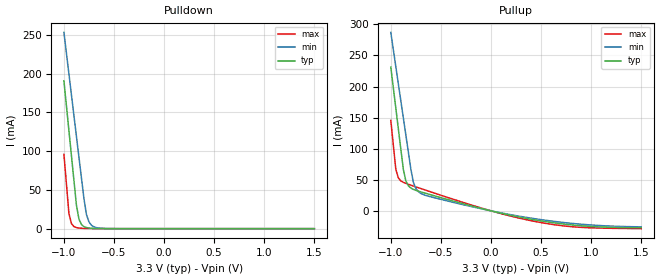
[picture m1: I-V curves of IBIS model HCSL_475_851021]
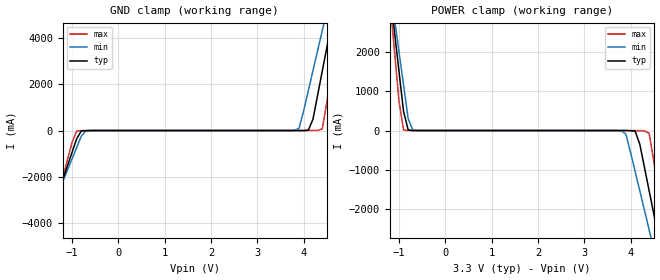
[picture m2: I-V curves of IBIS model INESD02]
|   This file is an IBIS representation of the   |
|   Integrated Circuit Systems, Inc.   |
|   ICS851021   |
[IBIS Ver]   4.0
[File name]   851021_rref_475.ibs
[File Rev]   1.0
[Date]   Dec 29 2006 | Last modified
|   Dec 29 2006 | Generated
[Source] Originated at Integrated Device Technology, Inc.
[Disclaimer]
IDT hereby grants the user of this IBIS model a non-exclusive,
nontransferable license to use this IBIS model under the following terms.
Before using this IBIS model, the user should read this license.
If the user does not accept these terms,  the IBIS model should be
returned to IDT within 30 days.
   The user is granted this license only to use the IBIS model and
is not granted rights to sell, load, rent, lease or license the IBIS
model in whole or in part, or in modified form to anyone other than
user. User may modify the IBIS model to suit its specific
applications but rights to derivative works and such modifications
shall belong to ICS.
   This IBIS model is provided on an "AS IS" basis and IDT makes
absolutely no warranty with respect to the information contained
herein. IDT DISCLAIMS AND CUSTOMER WAIVES ALL WARRANTIES, EXPRESS
OR IMPLIED, INCLUDING WARRANTIES OF MERCHANTABILITY OR FITNESS FOR
A PARTICULAR PURPOSE. The entire risk as to quality and performance
is with the Customer. ACCORDINGLY, IN NO EVENT SHALL THE COMPANY BE
LIABLE FOR ANY DAMAGES, WHETHER IN CONTRACT OR TORT,INCLUDING ANY
LOST PROFITS OR OTHER INCIDENTAL, CONSEQUENTIAL, EXEMPLARY, OR
PUNITIVE DAMAGES ARISING OUT OF THE USE OR APPLICATION OF THE IBIS
model provided in this package. Further, IDT reserves the right to
make changes without notice to any product herein to improve
reliability, function, or design. IDT does not convey any license
under patent rights or any other intellectual property rights,
including those of third parties.
   IDT is not obligated to provide maintenance or support
for the licensed IBIS model.
[Copyright]   Copyright 2006 by Integrated Device Technology, Inc.
[Component]   ICS851021AY
[Manufacturer] Integrated Device Technology, Inc.
[Package]
|TQFP 64 Pin lead+wire
|   typ   min   max
R_pkg   73.35m   65.90m   80.80m
L_pkg   2.615n   2.25n   2.98n
C_pkg   0.382p   0.366p   0.397p
[Pin] signal_name   model_name   R_pin   L_pin   C_pin
1   Q3   HCSL_475_851021   80.80m   2.98n   0.366p
2   nQ3   HCSL_475_851021   79.00m   2.81n   0.397p
3   VDD   POWER   74.90m   2.66n   0.390p
4   Q4   HCSL_475_851021   71.70m   2.54n   0.390p
5   nQ4   HCSL_475_851021   69.30m   2.44n   0.378p
6   GND   GND   67.60m   2.36n   0.373p
7   Q5   HCSL_475_851021   65.90m   2.30n   0.371p
8   nQ5   HCSL_475_851021   65.90m   2.25n   0.379p
9   VDD   POWER   65.90m   2.25n   0.379p
10   Q6   HCSL_475_851021   65.90m   2.30n   0.371p
11   nQ6   HCSL_475_851021   67.60m   2.36n   0.373p
12   Q7   HCSL_475_851021   69.30m   2.44n   0.378p
13   nQ7   HCSL_475_851021   71.70m   2.54n   0.390p
14   VDD   POWER   74.90m   2.66n   0.390p
15   Q8   HCSL_475_851021   79.00m   2.81n   0.397p
16   nQ8   HCSL_475_851021   80.80m   2.98n   0.366p
17   GND   GND   80.80m   2.98n   0.366p
|18  RREF   79.00m   2.81n   0.397p
19   Q9   HCSL_475_851021   74.90m   2.66n   0.390p
20   nQ9   HCSL_475_851021   71.70m   2.54n   0.390p
21   VDD   POWER   69.30m   2.44n   0.378p
22   Q10   HCSL_475_851021   67.60m   2.36n   0.373p
23   nQ10   HCSL_475_851021   65.90m   2.30n   0.371p
24   VDD   POWER   65.90m   2.25n   0.379p
25   VDDA   POWER   65.90m   2.25n   0.379p
|26  nc   65.90m   2.30n   0.371p
27   Q11   HCSL_475_851021   67.60m   2.36n   0.373p
28   nQ11   HCSL_475_851021   69.30m   2.44n   0.378p
29   VDD   POWER   71.70m   2.54n   0.390p
30   Q12   HCSL_475_851021   74.90m   2.66n   0.390p
31   nQ12   HCSL_475_851021   79.00m   2.81n   0.397p
32   GND   GND   80.80m   2.98n   0.366p
33   Q13   HCSL_475_851021   80.80m   2.98n   0.366p
34   nQ13   HCSL_475_851021   79.00m   2.81n   0.397p
35   VDD   POWER   74.90m   2.66n   0.390p
36   Q14   HCSL_475_851021   71.70m   2.54n   0.390p
37   nQ14   HCSL_475_851021   69.30m   2.44n   0.378p
38   Q15   HCSL_475_851021   67.60m   2.36n   0.373p
39   nQ15   HCSL_475_851021   65.90m   2.30n   0.371p
40   VDD   POWER   65.90m   2.25n   0.379p
41   Q16   HCSL_475_851021   65.90m   2.25n   0.379p
42   nQ16   HCSL_475_851021   65.90m   2.30n   0.371p
43   GND   GND   67.60m   2.36n   0.373p
44   Q17   HCSL_475_851021   69.30m   2.44n   0.378p
45   nQ17   HCSL_475_851021   71.70m   2.54n   0.390p
46   VDD   POWER   74.90m   2.66n   0.390p
47   Q18   HCSL_475_851021   79.00m   2.81n   0.397p
48   nQ18   HCSL_475_851021   80.80m   2.98n   0.366p
49   GND   GND   80.80m   2.98n   0.366p
50   CLK   INESD02   79.00m   2.81n   0.397p
51   nCLK   INESD02   74.90m   2.66n   0.390p
52   VDD   POWER   71.70m   2.54n   0.390p
53   Q19   HCSL_475_851021   69.30m   2.44n   0.378p
54   nQ19   HCSL_475_851021   67.60m   2.36n   0.373p
55   Q20   HCSL_475_851021   65.90m   2.30n   0.371p
56   nQ20   HCSL_475_851021   65.90m   2.25n   0.379p
57   VDD   POWER   65.90m   2.25n   0.379p
58   Q0   HCSL_475_851021   65.90m   2.30n   0.371p
59   nQ0   HCSL_475_851021   67.60m   2.36n   0.373p
60   Q1   HCSL_475_851021   69.30m   2.44n   0.378p
61   nQ1   HCSL_475_851021   71.70m   2.54n   0.390p
62   VDD   POWER   74.90m   2.66n   0.390p
63   Q2   HCSL_475_851021   79.00m   2.81n   0.397p
64   nQ2   HCSL_475_851021   80.80m   2.98n   0.366p
[Diff Pin]  inv_pin  vdiff tdelay_typ tdelay_min  tdelay_max
1   2   NA   0   0   0
4   5   NA   0   0   0
7   8   NA   0   0   0
10   11   NA   0   0   0
12   13   NA   0   0   0
15   16   NA   0   0   0
19   20   NA   0   0   0
22   23   NA   0   0   0
27   28   NA   0   0   0
30   31   NA   0   0   0
33   34   NA   0   0   0
36   37   NA   0   0   0
38   39   NA   0   0   0
41   42   NA   0   0   0
44   45   NA   0   0   0
47   48   NA   0   0   0
53   54   NA   0   0   0
55   56   NA   0   0   0
58   59   NA   0   0   0
60   61   NA   0   0   0
63   64   NA   0   0   0
|Input
50   51   NA   0   0   0
| Models and submodels in the file (2): HCSL_475_851021 (Output_ECL), INESD02 (Input)
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[Model]   HCSL_475_851021
Model_type  Output_ECL
Polarity   Non-Inverting
Vmeas = 0.3
Rref = 50
Cref = 0
Vref = 0
|Variable   typ   min   max
C_comp   2p   1.5p   2.5p
|Variable   typ   min   max
[Temperature Range]   25   0   70
|vddo
[Voltage Range]   3.3   3.135   3.465
|  Voltage   I(typ)   I(min)   I(max)
[Pullup]
-1V       231.3mA    287.2mA    145.6mA
-950mV    165.4mA    232.2mA    66.95mA
-925mV    132.5mA    204.7mA    53.21mA
-875mV    66.96mA    149.8mA    45.86mA
-850mV    48.22mA    122.3mA    44.19mA
-800mV    36.71mA    67.38mA    41.33mA
-775mV    34.58mA    46.1mA     39.96mA
-725mV    31.73mA    30.85mA    37.22mA
-250mV    10.23mA    8.861mA    12.13mA
475mV     -15.56mA   -13.58mA   -18.18mA
875mV     -23.69mA   -21.17mA   -26.35mA
1.5V      -27.26mA   -25.78mA   -28.68mA
[Pulldown]
-1V       190.7mA    253.2mA    96.06mA
-950mV    126.3mA    199.5mA    19.32mA
-925mV    94.15mA    172.6mA    6.574mA
-875mV    30.23mA    119mA      1.34mA
-850mV    12.34mA    92.17mA    792.6uA
-825mV    5.387mA    65.39mA    503.8uA
-800mV    2.598mA    38.64mA    322.7uA
-775mV    1.405mA    18.08mA    201.9uA
-750mV    838uA      8.675mA    122.1uA
-725mV    531uA      4.358mA    71.4uA
-550mV    17.95uA    128.7uA    737nA
1.5V      106.7pA    2.661nA    840.3fA
[Ramp]
|   typ   min   max
dV/dt_r   0.4V/0.2ns   0.35V/0.25ns   0.45V/0.2ns
dV/dt_f   0.4V/0.2ns   0.35V/0.25ns   0.45V/0.2ns
R_load =   50.0000
[Model]   INESD02
Model_type   Input
Polarity   Non-Inverting
Vinl = 1.4V
Vinh = 1.85V
|   typ   min   max
C_comp   2pF   1.5pF   2.5pF
|   typ   min   max
[Voltage range]  3.3V   3.15V   3.45V
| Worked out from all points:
|   GND clamp passes 1 mA (typ) near -0.60 V on its own axis
|   POWER clamp passes 1 mA (typ) near -0.70 V on its own axis
[GND_clamp]
|Voltage   I(typ)   I(min)   I(max)
-3.3V     -14.52A    -12.54A    -17.85A
-1.6V     -4.484A    -4.176A    -5.037A
-1.5V     -3.894A    -3.684A    -4.283A
-900mV    -353.5mA   -734.3mA   -21.75mA
-700mV    -3.477mA   -14.23mA   -2.542mA
3.9V      93.7uA     99.11mA    24.3nA
4.2V      488.4mA    2.584A     154.2uA
4.4V      2.557A     4.308A     69.78mA
4.6V      4.628A     6.034A     2.547A
4.7V      5.664A     6.897A     3.87A
4.8V      6.7A       7.76A      5.194A
6.6V      25.37A     23.32A     29.05A
[POWER_clamp]
|Voltage   I(typ)   I(min)   I(max)
-3.3V     25.37A     21.89A     31.23A
-1.2V     3.592A     3.748A     3.407A
-1.1V     2.557A     2.885A     2.084A
-900mV    488.4mA    1.162A     13.79mA
-700mV    784.1uA    13.23mA    69.84uA
3.8V      -170.4uA   -6.208mA   -212.5nA
4.1V      -17.77mA   -1.053A    -995.1uA
4.3V      -942.9mA   -2.036A    -8.426mA
4.4V      -1.533A    -2.528A    -72.77mA
4.6V      -2.713A    -3.512A    -1.531A
4.8V      -3.894A    -4.496A    -3.039A
6.6V      -14.52A    -13.36A    -16.61A
